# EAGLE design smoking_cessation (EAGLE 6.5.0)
TITLE: MONOXALYZE

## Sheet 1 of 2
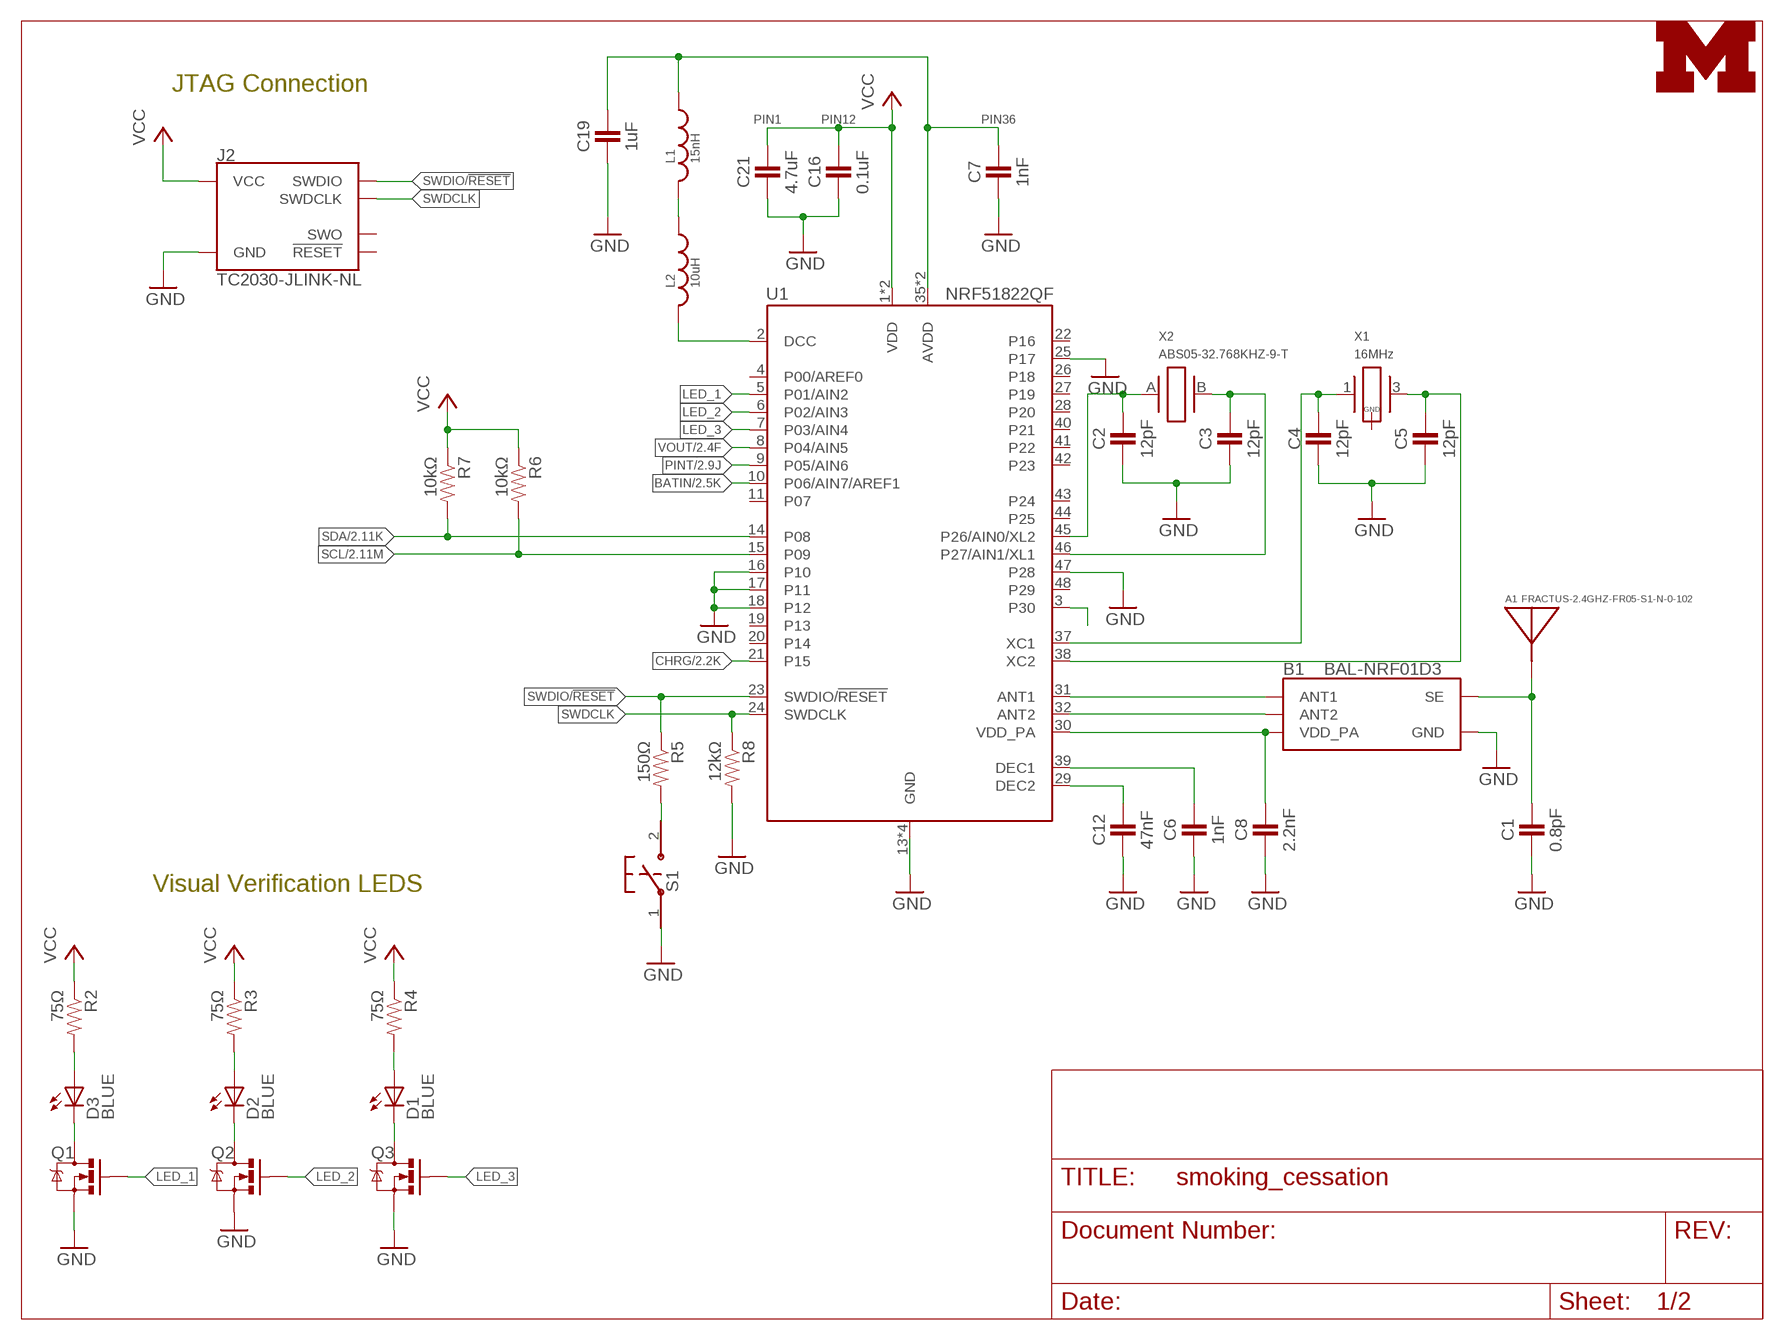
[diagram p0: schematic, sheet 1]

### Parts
A1  FRACTUS-2.4GHZ-FR05-S1-N-0-102  [FRACTUS-ANTENNA-FR05-S1-N-0-102]
B1  BAL-NRF01D3  [BAL-NRF01D3]
C1  0.8pF  CAPACITOR  [0402_CAP]
C2  12pF  CAPACITOR  [0402_CAP]
C3  12pF  CAPACITOR  [0402_CAP]
C4  12pF  CAPACITOR  [0402_CAP]
C5  12pF  CAPACITOR  [0402_CAP]
C6  1nF  CAPACITOR  [0402_CAP]
C7  1nF  CAPACITOR  [0402_CAP]
C8  2.2nF  CAPACITOR  [0402_CAP]
C12  47nF  CAPACITOR  [0402_CAP]
C16  0.1uF  CAPACITOR  [0402_CAP]
C19  1uF  CAPACITOR  [0402_CAP]
C21  4.7uF  CAPACITOR  [0402_CAP]
D1  BLUE  LED1206  [LED-1206]
D2  BLUE  LED1206  [LED-1206]
D3  BLUE  LED1206  [LED-1206]
J2  TC2030-JLINK-NL  [TC2030-IDC-NL]
L1  15nH  INDUCTOR0402  [0402_CAP]
L2  10uH  INDUCTOR0603  [0603_CAP]
LOGO1  UMICH_SOLID_TINY  [UMICH_SOLID_50MIL]
Q1  MOSFET-NCHANNELXFDN-3  [XFDFN-3]
Q2  MOSFET-NCHANNELXFDN-3  [XFDFN-3]
Q3  MOSFET-NCHANNELXFDN-3  [XFDFN-3]
R2  75Ω  RESISTOR0402_RES  [0402_RES]
R3  75Ω  RESISTOR0402_RES  [0402_RES]
R4  75Ω  RESISTOR0402_RES  [0402_RES]
R5  150Ω  RESISTOR0402_RES  [0402_RES]
R6  10kΩ  RESISTOR0402_RES  [0402_RES]
R7  10kΩ  RESISTOR0402_RES  [0402_RES]
R8  12kΩ  RESISTOR0402_RES  [0402_RES]
S1  B3U-1000P  [B3U-1000P]
U1  NRF51822QF  [QFN-48-6MM]
X1  16MHz  TXC-8Y  [TXC-8Y]
X2  ABS05-32.768KHZ-9-T  [ABS05]

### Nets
A0: C2.1 U1.45(P26/AIN0/XL2) X2.A
A1: C3.1 U1.46(P27/AIN1/XL1) X2.B
AVDD: C7.1 C19.1 L1.1 U1.35(AVDD) U1.36(AVDD)
BATIN: U1.10(P06/AIN7/AREF1) ; also sheet 2
CHRG: U1.21(P15) ; also sheet 2
DCC: L2.2 U1.2(DCC)
GND: B1.GND C1.2 C2.2 C3.2 C4.2 C5.2 C6.2 C7.2 C8.2 C12.2 C16.2 C19.2 C21.2 J2.5(GND) Q1.S Q2.S Q3.S R8.2 S1.1 U1.13(GND) U1.16(P10) U1.17(P11) U1.18(P12) U1.25(P17) U1.33(GND) U1.34(GND) U1.47(P28) U1.GND ; also sheet 2
LED_1: Q1.G U1.5(P01/AIN2)
LED_2: Q2.G U1.6(P02/AIN3)
LED_3: Q3.G U1.7(P03/AIN4)
N$5: B1.ANT1 U1.31(ANT1)
N$6: B1.ANT2 U1.32(ANT2)
N$7: D3.C Q1.D
N$9: D2.C Q2.D
N$10: D1.C Q3.D
N$11: A1.1(ANTENNA) B1.SE C1.1
N$14: L1.2 L2.1
N$16: C4.1 U1.37(XC1) X1.1
N$17: C5.1 U1.38(XC2) X1.3
N$18: C6.1 U1.39(DEC1)
N$19: C12.1 U1.29(DEC2)
N$20: D3.A R2.2
N$21: D2.A R3.2
N$22: D1.A R4.2
N$23: U1.3(P30)
N$24: R5.2 S1.2
PINT: U1.9(P05/AIN6) ; also sheet 2
SCL: R6.2 U1.15(P09) ; also sheet 2
SDA: R7.2 U1.14(P08) ; also sheet 2
SWDCLK: J2.4(SWDCLK) R8.1 U1.24(SWDCLK)
SWDIO/!RESET: J2.2(SWDIO) R5.1 U1.23(SWDIO/!RESET)
VCC: C16.1 C21.1 J2.1(VCC) R2.1 R3.1 R4.1 R6.1 R7.1 U1.1(VDD) U1.12(VDD) ; also sheet 2
VDD_PA: B1.VCC(VDD_PA) C8.1 U1.30(VDD_PA)
VOUT: U1.8(P04/AIN5) ; also sheet 2
Unconnected: J2.3(!RESET) J2.6(SWO) U1.4(P00/AREF0) U1.11(P07) U1.19(P13) U1.20(P14) U1.22(P16) U1.26(P18) U1.27(P19) U1.28(P20) U1.40(P21) U1.41(P22) U1.42(P23) U1.43(P24) U1.44(P25) U1.48(P29) X1.2(GND) X1.4(GND)

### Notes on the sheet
- JTAG Connection
- PIN1 | PIN12 | PIN36
- Visual Verification LEDS

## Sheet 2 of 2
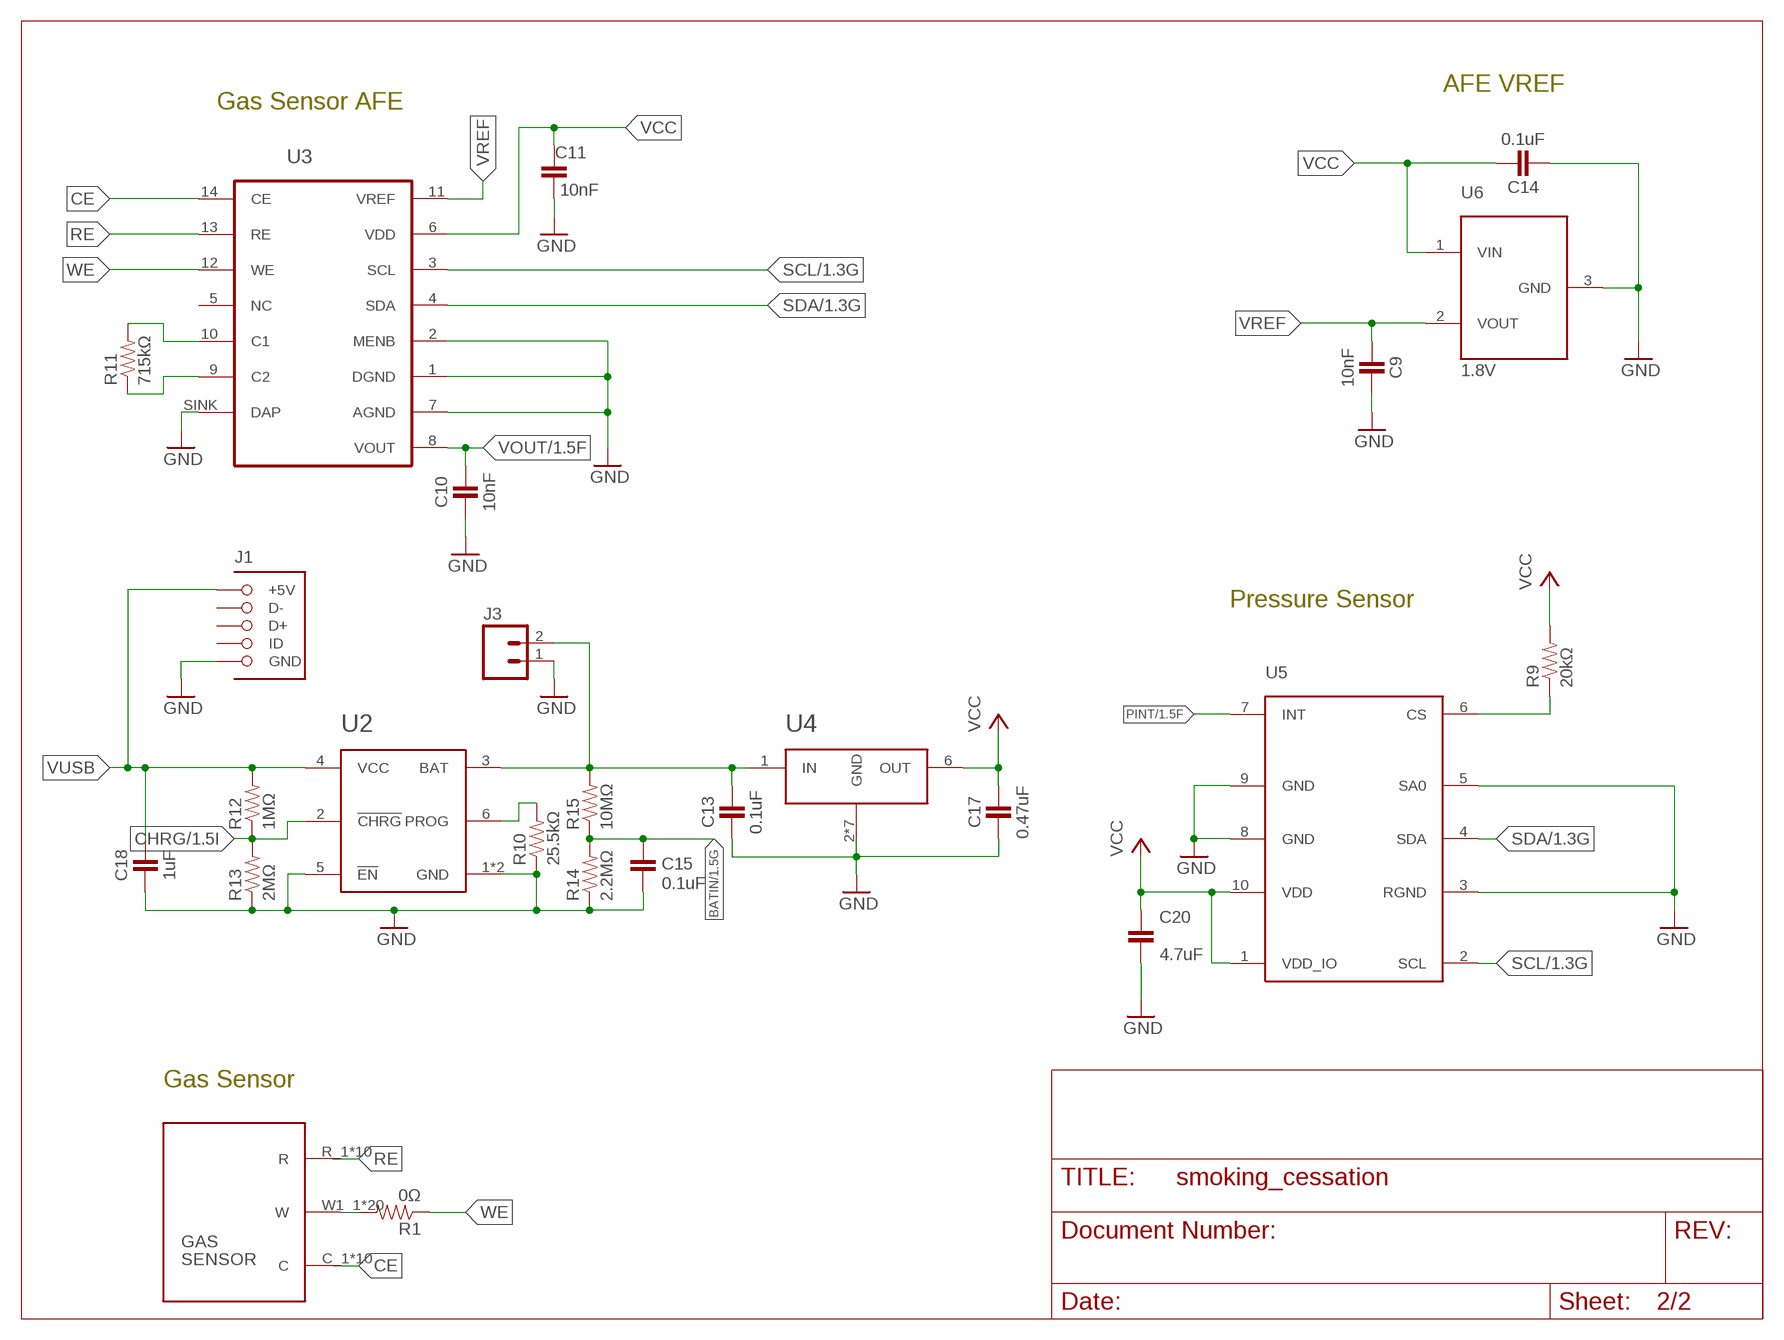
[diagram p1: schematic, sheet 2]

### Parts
C9  10nF  CAPACITOR  [0402_CAP]
C10  10nF  CAPACITOR  [0402_CAP]
C11  10nF  CAPACITOR  [0402_CAP]
C13  0.1uF  CAPACITOR  [0402_CAP]
C14  0.1uF  CAPACITOR  [0402_CAP]
C15  0.1uF  CAPACITOR  [0402_CAP]
C17  0.47uF  CAPACITOR  [0402_CAP]
C18  1uF  CAPACITOR  [0402_CAP]
C20  4.7uF  CAPACITOR  [0402_CAP]
J1  MOLEX_MICRO_USB_B_047346  [USB_MICRO_B-MOLEX-047346]
J3  M02PTH  [1X02]
R1  0Ω  RESISTOR0402_RES  [0402_RES]
R9  20kΩ  RESISTOR0402_RES  [0402_RES]
R10  25.5kΩ  RESISTOR0402_RES  [0402_RES]
R11  715kΩ  RESISTOR0402_RES  [0402_RES]
R12  1MΩ  RESISTOR0402_RES  [0402_RES]
R13  2MΩ  RESISTOR0402_RES  [0402_RES]
R14  2.2MΩ  RESISTOR0402_RES  [0402_RES]
R15  10MΩ  RESISTOR0402_RES  [0402_RES]
U2  LTC4065  [DFN-6/2MM]
U3  LMP91000  [WFDFN-14]
U4  TPS715AXX  [WDFN-6]
U5  LPS25H  [LPS25H]
U6  1.8V  ISL60002  [ISL60002]
U7  SPECSENSOR  [SPEC2]

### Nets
BATIN: C15.2 R14.2 R15.1 ; also sheet 1
CE: U3.14(CE) U7.C_1(C) U7.C_2(C) U7.C_3(C) U7.C_4(C) U7.C_5(C) U7.C_6(C) U7.C_7(C) U7.C_8(C) U7.C_9(C) U7.C_10(C)
CHRG: R12.1 R13.2 U2.2(!CHRG) ; also sheet 1
GND: C9.1 C10.2 C11.1 C13.2 C14.2 C15.1 C17.2 C18.2 C20.1 J1.GND J3.1 R10.1 R13.1 R14.1 U2.1(GND) U2.5(!EN) U2.7(GND) U3.1(DGND) U3.2(MENB) U3.7(AGND) U3.SINK(DAP) U4.2(GND) U4.3(GND) U4.4(GND) U4.5(GND) U4.TP2(GND) U4.TP3(GND) U4.TP(GND) U5.3(RGND) U5.5(SA0) U5.8(GND) U5.9(GND) U6.3(GND) ; also sheet 1
N$1: R1.2 U7.W1_1(W) U7.W1_2(W) U7.W1_3(W) U7.W1_4(W) U7.W1_5(W) U7.W1_6(W) U7.W1_7(W) U7.W1_8(W) U7.W1_9(W) U7.W1_10(W) U7.W2_1(W) U7.W2_2(W) U7.W2_3(W) U7.W2_4(W) U7.W2_5(W) U7.W2_6(W) U7.W2_7(W) U7.W2_8(W) U7.W2_9(W) U7.W2_10(W)
N$8: R11.2 U3.10(C1)
N$12: R11.1 U3.9(C2)
N$13: R10.2 U2.6(PROG)
N$15: R9.1 U5.6(CS)
PINT: U5.7(INT) ; also sheet 1
RE: U3.13(RE) U7.R_1(R) U7.R_2(R) U7.R_3(R) U7.R_4(R) U7.R_5(R) U7.R_6(R) U7.R_7(R) U7.R_8(R) U7.R_9(R) U7.R_10(R)
SCL: U3.3(SCL) U5.2(SCL) ; also sheet 1
SDA: U3.4(SDA) U5.4(SDA) ; also sheet 1
VBAT: C13.1 J3.2 R15.2 U2.3(BAT) U4.1(IN)
VCC: C11.2 C14.1 C17.1 C20.2 R9.2 U3.6(VDD) U4.6(OUT) U5.1(VDD_IO) U5.10(VDD) U6.1(VIN) ; also sheet 1
VOUT: C10.1 U3.8(VOUT) ; also sheet 1
VREF: C9.2 U3.11(VREF) U6.2(VOUT)
VUSB: C18.1 J1.VCC(+5V) R12.2 U2.4(VCC)
WE: R1.1 U3.12(WE)
Unconnected: J1.D+ J1.D- J1.ID U3.5(NC)

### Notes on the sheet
- AFE VREF
- Gas Sensor AFE
- Pressure Sensor
- Gas Sensor

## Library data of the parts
A1 = chips:FRACTUS-2.4GHZ-FR05-S1-N-0-102: Fractus Compact Reach XtendTM chip antenna is engineered specifically for Bluetooth,; RICHARDSON_RFPD: FR05-S1-N-0102B
B1 = chips:BAL-NRF01D3: 50 ohm nominal input / conjugate match balun to nRF51422-QFAA, nRF24LE1, nRF51822-QFAA/AB, with integrated harmonic filter; DIGIKEY: 497-13637-1-ND; MOUSER: 511-BAL-NRF01D3
C1 = passives:CAPACITOR: 0402 Capacitor; DIGIKEY: 490-6269-1-ND
C2-C5 = passives:CAPACITOR: 0402 Capacitor; DIGIKEY: 490-6197-1-ND
C6 C7 = passives:CAPACITOR: 0402 Capacitor; DIGIKEY: 490-1303-1-ND
C8 = passives:CAPACITOR: 0402 Capacitor; DIGIKEY: 490-5419-1-ND
C9-C11 C13-C15 C17 C18 C20 = passives:CAPACITOR: 0402 Capacitor
C12 = passives:CAPACITOR: 0402 Capacitor; DIGIKEY: 445-1264-1-ND
C16 = passives:CAPACITOR: 0402 Capacitor; DIGIKEY: 445-4952-1-ND
C19 = passives:CAPACITOR: 0402 Capacitor; DIGIKEY: 1276-1513-1-ND
C21 = passives:CAPACITOR: 0402 Capacitor; DIGIKEY: 445-5947-1-ND
D1-D3 = SparkFun-LED:LED: LEDs
J1 = connector:MOLEX_MICRO_USB_B_047346: Very tiny smd micro USB receptacle.; DIGIKEY: WM17141CT-ND
J2 = connector:TC2030-JLINK
J3 = SparkFun-Connectors:M02: Header 2
L1 = passives:INDUCTOR; DIGIKEY: 587-1521-1-ND
L2 = passives:INDUCTOR; DIGIKEY: 490-4025-1-ND
LOGO1 = logos:UMICH_SOLID
Q1-Q3 = fets:MOSFET-NCHANNEL: Generic NMOS footprint; DIGIKEY: DMN2400UFB4-7DICT-ND
R1 R9-R15 = passives:RESISTOR: Resistor
R2-R8 = passives:RESISTOR: Resistor; DIGIKEY: RHM12.0KCDCT-ND
S1 = switches:B3U: Switch; DIGIKEY: SW1020CT-ND
U1 = chips:NRF51822: Multiprotocol Bluetooth® 4.0 low energy/2.4 GHz RF SoC; DIGIKEY: 1490-1032-1-ND; MOUSER: 949-NRF51822-QFAB-R7
U2 = chips:LTC4065: LION/LIPO Battery Charging IC Low current; DIGIKEY: LTC4065LEDC#TRMPBF
U3 = chips:LMP91000: IC TI AFE for Gas Sensing; DIGIKEY: LMP91000SDE/NOPBCT-ND
U4 = chips:TPS715AXX: 80ma LDO Regulator. Very low quiescent current. Always active.; DIGIKEY: TPS715A33DRVR
U5 = chips:LPS25H: ST-Micro Piezoresistive pressure sensor; DIGIKEY: 497-15070-1-ND
U6 = chips:ISL60002: Low Power Voltage Reference SOT23-3; DIGIKEY: ISL60002BIH318Z-TKCT-ND
U7 = gas-sensor:SPECSENSOR: Three Electrod Gas Sensor
X1 = crystals:TXC-8Y: 2mmx1.6mm SMD Crystal; DIGIKEY: 887-2003-1-ND
X2 = crystals:ABS05-32.768KHZ: 32.768kHz Crystal; DIGIKEY: 535-11897-1-ND

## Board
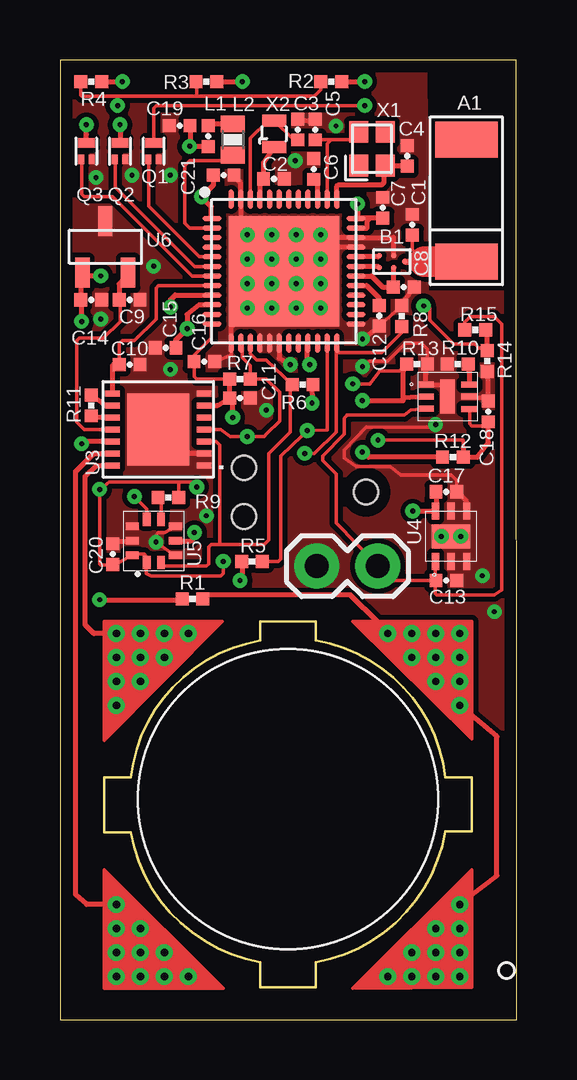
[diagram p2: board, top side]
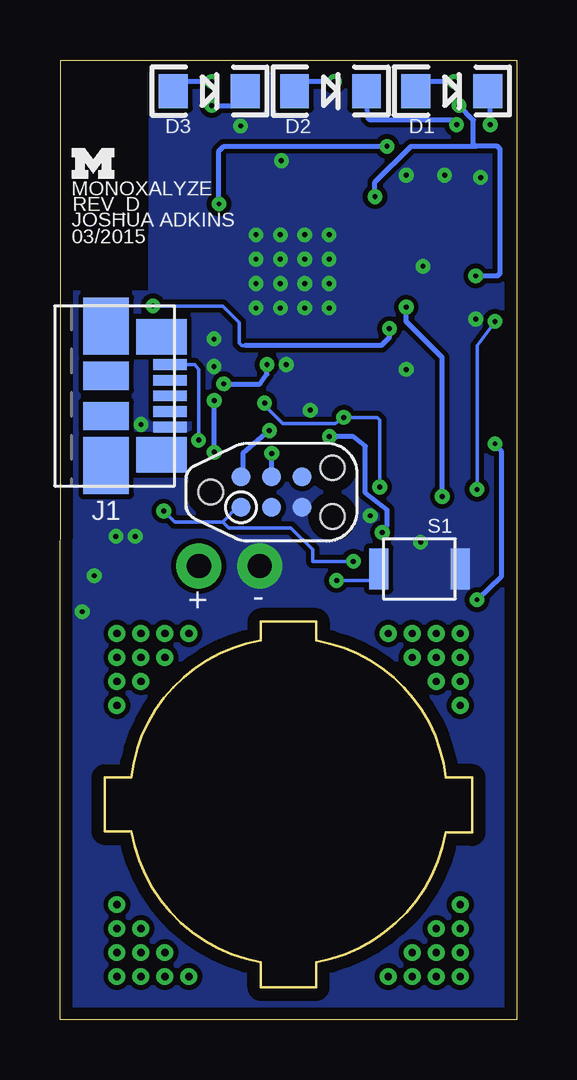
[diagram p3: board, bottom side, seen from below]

Size 19.02 x 40 mm. Coordinates in mm from the lower left corner, seen from the top.
Outline: 0,0 19.02,0 19,40 0,40 0,0
Copper layers (1*16): Top 0.0178mm / dielectric 59mil / Bottom 0.0178mm
Design rules "sunstone-2lyr_v1.0.0.3": minimum track width 6mil, minimum drill 14mil, track to track 6mil, track to pad 6mil, pad to pad 6mil, via to via 6mil, smd to smd 6mil, copper to edge 20mil, drill to drill 16mil, minimum pad ring 8mil, minimum via ring 8mil, stop-mask expansion 3mil, vias tented up to drill 0mil, thermal gap 10mil

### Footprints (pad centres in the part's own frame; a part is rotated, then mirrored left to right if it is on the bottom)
FRACTUS-ANTENNA-FR05-S1-N-0-102 = smd 1.5 x 2.6: 1 -2.55,0; 2 2.55,0
BAL-NRF01D3 = smd 0.22 x 0.22: ANT1 -0.537,-0.25; ANT2 -0.537,0.25; GND 0.069,0.25; SE 0.537,0; VCC 0.069,-0.25
0402_CAP = smd 0.536 x 0.546: 1 -0.433,0; 2 0.433,0
LED-1206 = smd 1.2 x 1.4: A -1.5,0; C 1.5,0
USB_MICRO_B-MOLEX-047346 = smd 1.38 x 0.45: D+ 2.66,0; D- 2.66,0.65; GND 2.66,-1.3; ID 2.66,-0.65; VCC 2.66,1.3 | smd 1.9 x 2.375: P$1 0,2.913; P$5 0,-2.913 | smd 2.1 x 1.475: P$2 2.3,2.462; P$6 2.3,-2.462 | smd 1.9 x 1.175: P$3 0,-0.838; P$4 0,0.838
TC2030-IDC-NL = smd 0.787 x 0.787: 1 -1.27,-0.635; 2 -1.27,0.635; 3 0,-0.635; 4 0,0.635; 5 1.27,-0.635; 6 1.27,0.635 | hole 1.016: -2.54,0; 2.54,1.016; 2.54,-1.016
1X02 = drill 1.016 pad 1.88: 1 0,0; 2 2.54,0
0603_CAP = smd 0.7 x 1: 1 -0.65,0; 2 0.65,0
XFDFN-3 = smd 0.4 x 0.7: D 0.35,0 | smd 0.4 x 0.25: G -0.35,0.215; S -0.35,-0.215
0402_RES = smd 0.536 x 0.546: 1 -0.433,0; 2 0.433,0
B3U-1000P = smd 0.8 x 1.7: 1 -1.7,0; 2 1.7,0
QFN-48-6MM = smd 0.8 x 0.203: 1 -3,2.2; 2 -3,1.8; 3 -3,1.4; 4 -3,1; 5 -3,0.6; 6 -3,0.2; 7 -3,-0.2; 8 -3,-0.6; 9 -3,-1; 10 -3,-1.4; 11 -3,-1.8; 12 -3,-2.2; 25 3,-2.2; 26 3,-1.8; 27 3,-1.4; 28 3,-1; 29 3,-0.6; 30 3,-0.2; 31 3,0.2; 32 3,0.6; 33 3,1; 34 3,1.4; 35 3,1.8; 36 3,2.2 | smd 0.203 x 0.8: 13 -2.2,-3; 14 -1.8,-3; 15 -1.4,-3; 16 -1,-3; 17 -0.6,-3; 18 -0.2,-3; 19 0.2,-3; 20 0.6,-3; 21 1,-3; 22 1.4,-3; 23 1.8,-3; 24 2.2,-3; 37 2.2,3; 38 1.8,3; 39 1.4,3; 40 1,3; 41 0.6,3; 42 0.2,3; 43 -0.2,3; 44 -0.6,3; 45 -1,3; 46 -1.4,3; 47 -1.8,3; 48 -2.2,3 | smd 4.6 x 4.6: GND 0,0
DFN-6/2MM = smd 0.25 x 0.675: 1 -0.5,-0.91; 2 0,-0.91; 3 0.5,-0.91; 4 0.51,0.91; 5 0,0.91; 6 -0.5,0.91 | smd 1.42 x 0.61: 7 0,0
WFDFN-14 = smd 0.25 x 0.6: 1 -1.5,-1.9; 2 -1,-1.9; 3 -0.5,-1.9; 4 0,-1.9; 5 0.5,-1.9; 6 1,-1.9; 7 1.5,-1.9; 8 1.5,1.9; 9 1,1.9; 10 0.5,1.9; 11 0,1.9; 12 -0.5,1.9; 13 -1,1.9; 14 -1.5,1.9 | smd 3 x 2.6: SINK 0,0
WDFN-6 = smd 0.3 x 0.7: 1 -0.65,-1.05; 2 0,-1.05; 3 0.65,-1.05; 4 0.65,1.05; 5 0,1.05; 6 -0.65,1.05 | drill 0.21 pad 0.406: TP -0.4,0; TP2 0.4,0 | smd 1.6 x 1: TP3 0,0
LPS25H = smd 0.32 x 0.55: 1 -0.3,-0.9; 2 0.3,-0.9; 6 0.3,0.9; 7 -0.3,0.9 | smd 0.55 x 0.32: 3 0.9,-0.6; 4 0.9,0; 5 0.9,0.6; 8 -0.9,0.6; 9 -0.9,0; 10 -0.9,-0.6
ISL60002 = smd 0.6 x 1.25: 1 -0.95,-1.08; 2 0.95,-1.08; 3 0,1.08
SPEC2 = drill 0.3: C_1 -7.15,7.15; C_2 -4.15,7.15; C_3 -5.15,7.15; C_4 -6.15,7.15; C_5 -7.15,5.15; C_6 -6.15,6.15; C_7 -5.15,6.15; C_8 -7.15,6.15; C_9 -6.15,5.15; C_10 -7.15,4.15; R_1 -7.15,-7.15; R_2 -6.15,-7.15; R_3 -5.15,-7.15; R_4 -4.15,-7.15; R_5 -5.15,-6.15; R_6 -6.15,-6.15; R_7 -7.15,-6.15; R_8 -6.15,-5.15; R_9 -7.15,-5.15; R_10 -7.15,-4.15; W1_1 7.15,7.15; W1_2 6.15,7.15; W1_3 5.15,7.15; W1_4 4.15,7.15; W1_5 7.15,6.15; W1_6 6.15,6.15; W1_7 5.15,6.15; W1_8 7.15,5.15; W1_9 6.15,5.15; W1_10 7.15,4.15; W2_1 7.15,-7.15; W2_2 6.15,-7.15; W2_3 5.15,-7.15; W2_4 4.15,-7.15; W2_5 7.15,-6.15; W2_6 6.15,-6.15; W2_7 5.15,-6.15; W2_8 7.15,-5.15; W2_9 6.15,-5.15; W2_10 7.15,-4.15
TXC-8Y = smd 0.9 x 0.8: 1 -0.7,-0.55; 2 0.7,-0.55; 3 0.7,0.55; 4 -0.7,0.55
ABS05 = smd 0.5 x 1: A -0.55,0; B 0.55,0

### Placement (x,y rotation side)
A1  16.93,34.13 90 top
B1  13.83,31.59 0 top
C1  14.68,33.13 90 top
C2  8.91,35.04 0 top
C3  9.9,37.1 90 top
C4  14.46,36 90 top
C5  10.63,37.1 90 top
C6  10.58,35.45 90 top
C7  13.46,33.84 90 top
C8  14.32,30.54 0 top
C9  2.9,30 180 top
C10  2.9,27.3 0 top
C11  7.5,25.9 180 top
C12  13.3,29.33 270 top
C13  16.1,18.3 0 top
C14  1.3,30 0 top
C15  4.4,28 0 top
C16  6.02,27.42 0 top
C17  16.1,22 0 top
C18  17.85,25.35 90 top
C19  4.98,37.27 180 top
C20  2.2,19.4 270 top
C21  6.82,35.2 0 top
D1  2.7,38.7 0 bottom
D2  7.75,38.7 0 bottom
D3  12.8,38.7 0 bottom
J1  17.1,26 0 bottom
J2  10.21,21.99 0 bottom
J3  10.7,18.9 0 top
L1  6.18,36.82 90 top
L2  7.2,36.68 270 top
LOGO1  17.64,35.68 0 bottom
Q1  3.9,36.2 90 top
Q2  2.5,36.2 90 top
Q3  1.1,36.2 90 top
R1  5.52,17.54 0 top
R2  11.3,39.1 0 top
R3  6.1,39.1 0 top
R4  1.3,39.1 0 top
R5  8,19.1 180 top
R6  10.11,26.47 180 top
R7  7.5,26.7 0 top
R8  14.24,29.32 90 top
R9  4.51,21.77 0 top
R10  16.57,27.33 0 top
R11  1.3,25.6 270 top
R12  16.37,23.45 0 top
R13  14.88,27.33 180 top
R14  17.8,27.45 90 top
R15  17.3,28.75 180 top
S1  4.05,18.79 180 bottom
U1  9.33,31.19 0 top
U2  16.15,25.96 270 top
U3  4.09,24.6 90 top
U4  16.29,20.14 0 top
U5  3.91,19.96 0 top
U6  1.89,32.21 0 top
U7  9.5,8.94 0 top
X1  13,36.3 90 top
X2  8.93,36.92 90 top

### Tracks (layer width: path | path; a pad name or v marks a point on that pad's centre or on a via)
A0
  Top 0.203: U1.45 8.33,34.89 C2.1 8.48,35.73 X2.A
A1
  Top 0.152: U1.46 7.93,36.73 8.67,37.47 X2.B 9.73,36.67 C3.1
AVDD  (via drill 0.2)
  Top 0.203: C7.1 12.9,33.4 | 12.9,33.4 12.34,33.4 U1.36 12.4,33.46 v12.4,34 | U1.35 12.79,32.99 12.8,33 12.8,33.3 12.9,33.4 | L1.1 6.28,36.4 v5.4,36.4 5.42,36.42 C19.1
  Bottom 0.203: v12.4,34 12.4,36.2 12.2,36.4 v5.4,36.4
BATIN  (via drill 0.2)
  Top 0.152: v15.15,29.75 15.35,29.75 15.4,29.65 15.4,29.15 16.4,28.15 17.3,28.15 17.45,28 17.77,28 R14.2
  Top 0.203: U1.10 5.8,29.8 5.3,29.4 v5.3,28.8 4.83,28.33 C15.2 | R14.2 17.8,28.43 R15.1
  Bottom 0.152: 11.3,28.1 11.45,28.1 11.55,28.2 11.55,29.05 12.25,29.75 v15.15,29.75
  Bottom 0.203: 11.3,28.1 5.63,28.1 5.3,28.43 v5.3,28.8
CE
  Top 0.152: 2.29,23.1 U3.14
  Top 0.203: U7.C_1 1.41,16.09 1.05,16.45 1.05,22.65 1.5,23.1 2.29,23.1
  Top 0.406: U7.C_4 U7.C_3 | U7.C_3 U7.C_7 | U7.C_3 U7.C_2 | U7.C_2 U7.C_6 U7.C_9 | U7.C_2 U7.C_1 U7.C_5 U7.C_8 U7.C_10
CHRG  (via drill 0.2)
  Top 0.152: v12.2,26.5 12.9,26.5 13.33,27.03 14.14,27.03 R13.2
  Top 0.203: U2.2 14.29,25.91 14.3,25.8 | 14.3,25.8 14.3,27.02 R13.2 | v10.4,27.3 10.3,27.4 10.3,28.16 U1.21 | R12.1 12.85,23.45 v12.6,23.65 | v12.6,25.8 14.3,25.8
  Bottom 0.203: v12.6,23.65 v12.6,25.8 | v12.2,26.5 10.7,26.5 10.4,26.9 v10.4,27.3
DCC
  Top 0.152: U1.2 5.41,32.99 5.2,33.2 5.2,35.6 5.4,35.8 6.97,35.8
  Top 0.203: 7.09,35.92 L2.2 6.97,35.8
GND  (via drill 0.2)
  Top 0.152: C16.2 7.13,27.7 U1.13 | C12.2 R8.2 | 4.74,19.36 v4,19.9 4,20.2 4.1,20.3 4.36,20.3 U5.5 | R13.1 15.31,27.94 15.05,28.2 14.4,28.2 13.65,27.45 12.9,27.45 12.72,27.27 v12.61,27.22 | C17.2 16.53,22.47 16.3,22.7 14.2,22.7 13.75,23.05 12.35,23.05 11.85,23.4 11.85,23.75 12.75,24.7 15.55,24.7 v15.65,24.8
  Top 0.203: U1.13 7.13,28.86 v7.81,29.66 | B1.GND 13.9,32.59 U1.34 11.1,32.59 v10.86,32.71 11.5,32.19 U1.33 | v7.81,31.7 v7.81,32.71 7.53,32.99 U1.47 7.5,34.23 7.5,34.9 7.25,35.15 C21.2 | v12.61,28.37 12.77,28.47 C12.2 | R8.2 14.24,29.82 C8.2 | v8.82,31.7 v8.83,31.7 U1.GND | C3.2 10.63,37.43 C5.2 10.77,37.44 | U2.5 17.86,25.91 C18.2 R14.1 | 15.24,26.91 R13.1 15.24,26.94 15.24,26.91 | 15.95,26.41 16,26.41 16,26.45 U2.1 15.24,26.91 | C20.1 2.34,19.93 U5.9 | U5.3 4.74,19.36 | U3.2 5.2,23.6 5.1,23.7 4.79,24 U3.SINK | U1.18 9.13,27.57 v9.6,27.3 | U4.4 16.94,21.59 C17.2 | U5.5 4.7,20.5 4.76,20.56 4.66,20.56
  other vias: 9.84,31.7 9.84,30.68 9.84,29.66 9.84,32.71 10.86,31.7 10.86,30.68 10.86,29.66 8.83,29.66 8.83,30.68 8.83,32.71 7.81,30.68 9.8,35.8 17.6,18.5 18.1,17 3.9,31.4 4.6,35.2 3,35.2 1.5,35.1 1.7,29.2 8.6,25.4 4.6,27.1 11.5,37.25 6.1,21
  pour Top (isolate 0.203, no thermals): 0,40 15.2,40 15.25,30.3 19.1,30.3 19,0 0,0
  pour Bottom (isolate 0.203, no thermals): 19,0 19.1,30.3 15.25,30.3 15.2,40 0,40 0,0
LED_1
  Top 0.152: U1.5 5.81,31.79 3.7,33.9 3.7,35.84
  Top 0.203: 3.7,35.84 Q1.G
LED_2
  Top 0.152: U1.6 5.61,31.39 2.3,34.7 2.3,35.84
  Top 0.203: 2.3,35.84 Q2.G
LED_3
  Top 0.152: U1.7 5.51,30.99 2.2,34.3 1,34.3 0.9,34.4 0.9,35.83
  Top 0.203: 0.9,35.83 Q3.G
N$1
  Top 0.152: U7.W2_10 | U7.W1_4 13.26,16.54 | 6.09,17.7 R1.2
  Top 0.203: U7.W2_10 18.2,6 18.2,11.79 U7.W1_10 | 13.26,16.54 12.1,17.7 6.09,17.7
  Top 0.406: U7.W1_4 U7.W1_3 U7.W1_2 | U7.W1_2 U7.W1_1 U7.W1_5 U7.W1_8 U7.W1_10 | U7.W1_2 U7.W1_6 | U7.W1_7 U7.W1_6 | U7.W1_6 U7.W1_9 | U7.W2_4 U7.W2_3 U7.W2_2 U7.W2_6 | U7.W2_7 U7.W2_6 | U7.W2_6 U7.W2_5 | U7.W2_1 U7.W2_5 | U7.W2_5 U7.W2_8 | U7.W2_9 U7.W2_8 | U7.W2_8 U7.W2_10
N$5
  Top 0.203: B1.ANT1 13.24,31.39 U1.31
N$6
  Top 0.203: B1.ANT2 13.24,31.79 U1.32
N$7  (via drill 0.2)
  Top 0.152: Q1.D 3.9,38 4,38.1 v12.7,38.1
  Bottom 0.203: v12.7,38.1 11.7,38.1 11.7,38.5 11.6,38.5 D3.C
N$8
  Top 0.203: U3.10 1.3,25.1 R11.2
N$9  (via drill 0.2)
  Top 0.203: v2.5,37.3 Q2.D
  Bottom 0.203: v2.5,37.3 2.5,37.4 2.7,37.5 6.1,37.5 6.2,37.6 D2.C
N$10  (via drill 0.2)
  Top 0.203: Q3.D 1.1,36.9 v1.1,37.3
  Bottom 0.203: 0.9,38.8 D1.C 1.1,38.3 v1.1,37.3
N$11
  Top 0.152: C1.1 14.68,32.09 15.18,31.59
  Top 0.203: 14.71,31.59 15.18,31.59
  Top 0.254: B1.SE 14.71,31.59
  Top 0.762: 17.32,31.59 A1.1
  Top 1.27: 15.18,31.59 17.32,31.59
N$12
  Top 0.203: U3.9 1.9,25.6 R11.1
N$13
  Top 0.203: U2.6 17.06,26.97 R10.2
N$14
  Top 0.203: L2.1 6.37,37.33 L1.2
N$15
  Top 0.152: U5.6 4.21,21.7
  Top 0.203: 4.21,21.7 R9.1
N$16
  Top 0.203: C4.1 13.91,35.58 X1.1 13.5,35.44 13.5,34.9 13.4,34.8 11.6,34.8 11.53,34.73 U1.37
N$17
  Top 0.152: C5.1 11.3,36.67 | 11.3,36.67 12.27,36.67 | U1.38 11.13,36.5 11.3,36.67
  Top 0.203: 12.27,36.67 X1.3
N$18
  Top 0.203: U1.39 10.73,34.97 C6.1
N$19
  Top 0.203: U1.29 12.77,30.59 13.3,30.07 C12.1
N$20  (via drill 0.2)
  Top 0.203: R2.2 v12.7,39.1
  Bottom 0.203: 14.34,38.9 D3.A 13.9,39.1 v12.7,39.1
N$21  (via drill 0.2)
  Top 0.203: R3.2 v7.6,39.1
  Bottom 0.203: 9.34,38.9 D2.A 8.8,39.1 v7.6,39.1
N$22  (via drill 0.2)
  Top 0.203: R4.2 v2.6,39.1
  Bottom 0.203: 3.89,38.9 D1.A 3.6,39.1 v2.6,39.1
N$24  (via drill 0.2)
  Top 0.203: R5.2 7.6,18.9 7.6,18.4 v7.5,18.3
  Bottom 0.152: 5.9,18.3 v7.5,18.3
  Bottom 0.203: S1.2 5.85,18.35 5.9,18.3
PINT  (via drill 0.2)
  Top 0.152: U5.7 3.61,21.29 v3.1,21.8
  Top 0.203: v4.6,29.7 4.6,30 4.8,30.2 U1.9
  Bottom 0.203: v3.1,21.8 3.1,27.6 4.6,29.1 v4.6,29.7
RE
  Top 0.152: U3.13
  Top 0.203: U7.R_10 1.11,4.79 0.65,5.2 0.65,22.85 1.4,23.6 U3.13
  Top 0.406: U7.R_4 U7.R_3 U7.R_5 U7.R_6 | U7.R_1 U7.R_2 U7.R_6 | U7.R_6 U7.R_8 U7.R_9 | U7.R_7 U7.R_9 | U7.R_9 U7.R_10
SCL
  Top 0.152: U5.2 4.21,19.19 4.3,18.9 6.1,18.9 6.2,19 6.2,19.7 6.3,19.8 6.65,19.8 | 6.65,19.8 8.5,19.8 8.7,20 8.7,23.6 9.6,24.5 9.6,26.45 R6.2 8.6,27.5 8.2,27.5 7.93,27.77 U1.15 | U3.3 6.5,24.1 6.65,23.95 6.65,19.8
  Top 0.203: U3.3
SDA  (via drill 0.2)
  Top 0.152: U3.4 6.7,24.6 7.1,24.3 v7.8,24.3 8.5,24.3 8.6,24.4 9.15,24.95 9.15,26.15 8.6,26.7 R7.2 7.93,27.27 7.6,27.6 7.6,28.13 U1.14
  Top 0.203: U5.4 5.46,19.96 5.6,20.1 v5.6,20.3
  Bottom 0.203: v5.6,20.3 5.6,20.4 5.4,20.6 5.4,21.25 6.3,21.95 6.3,23.9 6.8,24.3 7.5,24.3 v7.8,24.3
SWDCLK  (via drill 0.2)
  Top 0.152: R8.1 14.24,28.64 13.4,27.8 11.53,27.8 U1.24 11.5,28.01 11.5,24.5 10.6,23.6 v10.2,23.6
  Bottom 0.203: J2.4 10.21,23.29 v10.2,23.6
SWDIO/!RESET  (via drill 0.2)
  Top 0.152: R5.1 9.1,19.1 9.2,19.2 9.2,23.5 10.1,24.35 v10.3,24.55 11.13,24.58 U1.23
  Bottom 0.203: v10.3,24.55 11.4,23.6 11.4,22.75 J2.2
VBAT
  Top 0.152: R15.2 16.87,29.07 17.1,29.3 18.1,29.3 18.4,29 18.4,17.9 18.1,17.7 15.7,17.7 15.64,17.76 15.64,18.32 U4.1 | U2.3 14.61,25.41 14.35,25.2 11.95,25.2 11.85,25.05 11.85,24.4 10.95,23.5 10.95,23.3 11.5,22.75 11.5,20.7 13.19,18.96 J3.2 13.85,18.3 C13.1
  Top 0.203: 15.64,18.32 C13.1
VCC  (via drill 0.2)
  Top 0.152: R4.1 0.87,38.53 0.9,38.5 2.4,38.5 | 5.7,38.5 5.7,39.27 | 5.7,38.5 10.6,38.5 10.87,38.77 R2.1 | 5.7,38.5 2.4,38.5 | 2.4,38.5 v2.4,38.1 | U5.1 3.61,19.29 3.5,19.4 3.06,19.4 | U5.10 2.29,18.96 1.69,18.96 1.65,19 v1.65,22.1 2.05,22.4 5,22.4 | R9.2 4.95,22.35 5,22.4 | 5,22.4 5.5,22.4 v5.7,22.2 | v6.8,19.1 6.8,18.6 6.7,18.5 3.8,18.5 3.6,18.6 3.6,19.24 | R7.1 5.7,26.7 5.6,26.8 5.6,27.4 C16.1 5.58,27.68 6.3,28.4 6.3,28.96 U1.12
  Top 0.203: U1.1 6.31,33.39 6.31,33.89 v5.9,34.3 6.39,34.79 C21.1 | 5.7,39.27 R3.1 | R2.1 10.87,38.97 | 0.74,31.5 U6.1 0.87,31 | v1.7,31 0.87,31 | 0.87,31 0.87,30.3 C14.1 0.9,29.97 v0.9,29.1 | C11.2 R7.1 | U3.6 6.57,25.6 C11.2 | 3.06,19.4 U5.10 | 2.29,18.96 C20.2 | v7.2,25.1 7.2,25.93 C11.2 | R6.1 10.49,26.49 v10.5,25.7 | C17.1 15.67,21.22 U4.6 v14.7,21.2 | 3.6,19.24 U5.1
  Bottom 0.152: v5.7,22.2 5.7,25 5.8,25.1 v7.2,25.1 7.55,24.85 9.75,24.85 10.5,25.6 v10.5,25.7 | 11.6,21.4 12.25,20.75 | 12.25,20.75 14.25,20.75 v14.7,21.2 | v1.65,22.1 1.65,28.1 v0.9,29.1 | v6.8,19.1 8.5,19.1 8.5,19.6 9.4,20.5 12,20.5 12.25,20.75
  Bottom 0.203: 1.7,36.4 0.8,36.4 0.7,36.3 0.7,31.1 0.8,31 v1.7,31 | 1.7,36.4 1.8,36.5 1.8,37.5 v2.4,38.1 | v5.9,34.3 5.9,34.9 4.4,36.4 1.7,36.4 | J2.1 11.6,21.4
VDD_PA
  Top 0.203: U1.30 12.98,30.99 13.44,30.54 C8.1 B1.VCC
VOUT
  Top 0.152: C10.1 2.47,28.17 2.6,28.3 3.1,28.3 4,29.2 4,30.5 4.1,30.6 U1.8
  Top 0.203: U3.8 2.2,27.1 2.2,27.3 2.3,27.3 C10.1 | U1.8
VREF
  Top 0.152: U3.11 1,24.6 0.7,24.9 0.7,28.3 0.8,28.4 1.8,28.4 2.5,29.1 2.5,29.97
  Top 0.203: U6.2 2.47,30.66 C9.2 2.5,29.97
VUSB  (via drill 0.2)
  Top 0.152: U2.4 17.06,24.84 17.15,24.75 17.83,24.75 C18.1 | 16.8,23.84 16.8,24.15 v13.25,24.15
  Top 0.203: 16.8,23.84 R12.2 17.4,23.45 17.85,24.05 C18.1
  Bottom 0.152: J1.VCC 13.4,27.3 13.25,27.1 v13.25,24.15
WE  (via drill 0.2)
  Top 0.203: U3.12 1,24.1 v0.9,24 | v1.65,17.5 5.15,17.5 R1.1
  Bottom 0.203: v0.9,24 0.65,23.7 0.65,18.45 v1.65,17.5

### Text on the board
bNames: REV_D | MONOXALYZE | JOSHUA ADKINS | 03/2015 | - | +

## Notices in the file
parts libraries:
SparkFun-LED: Licensing: CC v3.0 Share-Alike You are welcome to use this library for commercial purposes.
